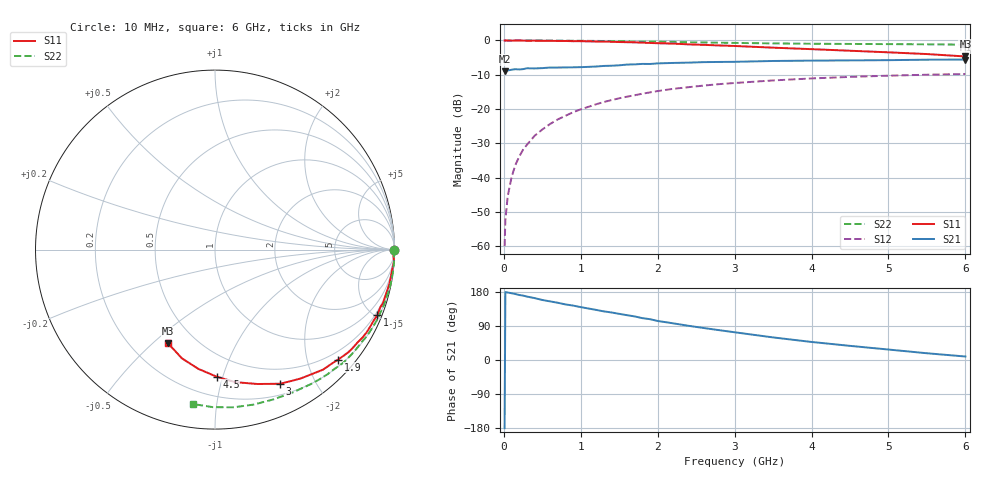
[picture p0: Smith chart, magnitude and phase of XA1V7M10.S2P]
! SIEMENS Discrete & RF Semiconductors
! BFY180
! Si NPN RF Bipolar Junction Transistor in MICRO-X
! VCE = 1.75 V  IC = 0.1 mA
! Common Emitter S-Parameters:  May  1997
# GHz  S  MA  R  50
!  f  S11  S21  S12  S22
! GHz  MAG  ANG  MAG  ANG  MAG  ANG  MAG  ANG
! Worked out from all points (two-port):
!   36 points, 10 MHz to 6 GHz, reference 50 ohm
!   highest |S21| = -5.56 dB at 6 GHz (marker M1); lowest = -9.0 dB at 10 MHz (marker M2)
!   |S21| within 3 dB of the highest: 94.99 MHz to end of sweep
!   lowest |S11| = -4.7 dB at 6 GHz (marker M3), VSWR 3.81, Z = 17.7 - j28 ohm
!   |S11| at or under -10 dB: nowhere
!   |S22| runs from -1.2 to 0.0 dB; largest |S21 - S12| = 0.39
!   S11 on the Smith chart (normalised r, x): 10 MHz: open; 1 GHz: 0.34, -5.15; 1.9 GHz: 0.32, -2.58; 3 GHz: 0.32, -1.55; 4.5 GHz: 0.34, -0.95; 6 GHz: 0.35, -0.56
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0.01  0.9956 -0.1  0.354 -179.9  0.001 95.4  0.9988 -0.2
0.02  0.9964 -0.5  0.367 179.4  0.0024 88.0  0.9999 -0.5
0.05  0.995 -0.7  0.365 178.1  0.0053 85.7  1 -1.0
0.1  0.9943 -2.1  0.374 176.2  0.0101 89.6  0.9974 -1.9
0.15  0.999 -3.4  0.381 174.1  0.0153 87.7  0.9999 -2.9
0.25  0.9948 -5.6  0.382 170.0  0.0256 85.2  0.9999 -4.8
0.4  0.9916 -8.9  0.391 163.3  0.0407 82.5  0.9991 -7.7
0.6  0.9865 -13.3  0.403 154.7  0.0604 78.1  0.9967 -11.5
0.7  0.9833 -15.6  0.403 151.1  0.0705 75.7  0.9948 -13.5
1  0.9755 -21.9  0.408 139.5  0.099 69.5  0.9897 -19.2
1.1  0.9686 -24.1  0.412 135.9  0.1077 67.6  0.986 -21.0
1.4  0.9565 -30.9  0.428 125.4  0.1351 61.4  0.978 -26.8
1.8  0.9287 -39.6  0.455 110.5  0.1674 53.7  0.9639 -34.1
1.9  0.9198 -41.8  0.454 107.7  0.1748 51.7  0.9613 -35.9
2.2  0.8999 -48.0  0.47 96.8  0.1969 45.9  0.9537 -41.3
2.6  0.8625 -56.3  0.483 84.4  0.22 38.8  0.9356 -47.9
3  0.8308 -64.1  0.488 73.2  0.2397 31.9  0.9206 -54.4
3.5  0.7852 -72.5  0.502 59.6  0.2612 24.6  0.9059 -61.6
4  0.7467 -81.4  0.508 47.6  0.2792 17.4  0.8957 -68.9
4.5  0.7079 -89.3  0.512 37.3  0.2942 10.7  0.8898 -76.1
5.5  0.6334 -106.9  0.524 17.8  0.3164 -2.4  0.8778 -90.8
6  0.584 -116.6  0.527 9.2  0.324 -9.1  0.869 -98.1
